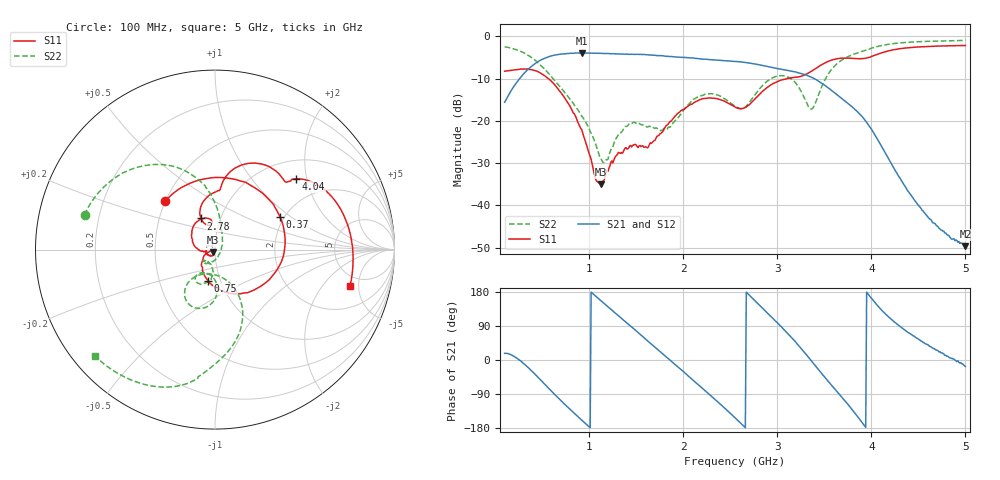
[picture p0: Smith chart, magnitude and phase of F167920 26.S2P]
!  2-Port S-parameters saved by WinCal
! VAR MeasName=S-Parameters (CALIBRATED_DATA) read from VNA (N5242A)
! VAR MeasDate=2016-11-22 9:56:27
! VAR NAME=F167920 26
! VAR FILENAME=F167920 26.S2P
! VAR DATE=2016-11-22 9:56:27
! VAR PHYS_PORTS=1,2
# Hz S DB R 50
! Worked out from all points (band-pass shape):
!   491 points, 100 MHz to 5 GHz, reference 50 ohm
!   highest |S21| = -3.91 dB at 920 MHz (marker M1); lowest = -49.7 dB at 5 GHz (marker M2)
!   |S21| within 3 dB of the highest: 396.6 MHz to 2.847 GHz (2.451 GHz wide, 151 % of centre)
!   lowest |S11| = -35.0 dB at 1.12 GHz (marker M3), VSWR 1.04, Z = 49 - j1.47 ohm
!   |S11| at or under -10 dB: 566.2 MHz to 3.101 GHz (2.535 GHz wide, 138 % of centre)
!   |S22| runs from -29.9 to -1.0 dB; largest |S21 - S12| = 0.0012
!   S11 on the Smith chart (normalised r, x): 100 MHz: 0.50, +0.32; 370 MHz: 1.90, +0.82; 750 MHz: 0.87, -0.31; 2.78 GHz: 0.81, +0.29; 4.04 GHz: 1.40, +1.73; 5 GHz: 3.86, -3.97
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1e8  -8.25 135.7  -15.60 17.5  -15.61 17.5  -2.47 165.1
2.3e8  -7.87 81.2  -10.85 4.7  -10.85 4.8  -3.20 145.9
3.7e8  -7.85 26.5  -7.40 -24.6  -7.40 -24.5  -4.76 124.9
5.6e8  -9.93 -42.3  -4.90 -72.4  -4.90 -72.4  -8.58 100.4
7.5e8  -14.99 -102.2  -4.10 -119.5  -4.09 -119.5  -13.55 85.1
9.2e8  -22.07 -146.0  -3.91 -158.6  -3.91 -158.6  -18.92 71.4
1.12e9  -35.02 -122.2  -4.02 157.3  -4.01 157.3  -28.75 10.7
1.18e9  -32.06 -102.9  -4.07 144.5  -4.07 144.5  -29.17 -42.0
1.43e9  -25.92 -144.0  -4.26 91.6  -4.26 91.6  -20.58 -122.8
1.74e9  -23.46 -172.4  -4.55 25.0  -4.55 25.0  -22.14 -126.9
1.94e9  -18.25 166.6  -4.92 -17.6  -4.92 -17.7  -19.43 -97.9
2.17e9  -15.05 133.1  -5.31 -67.7  -5.31 -67.8  -14.21 -106.4
2.36e9  -14.74 106.0  -5.64 -109.0  -5.65 -109.0  -13.87 -121.9
2.55e9  -16.75 96.7  -5.93 -152.2  -5.93 -152.2  -16.53 -120.0
2.78e9  -14.39 114.2  -6.61 152.1  -6.62 152.0  -13.30 -86.3
3.06e9  -10.24 94.8  -7.87 83.3  -7.89 83.4  -9.32 -111.9
3.37e9  -8.16 82.8  -9.74 -4.6  -9.75 -4.6  -17.12 -92.0
3.62e9  -5.37 62.7  -13.54 -79.2  -13.57 -79.0  -6.77 -71.7
4.04e9  -4.45 41.1  -23.39 151.2  -23.42 151.4  -2.54 -99.9
4.19e9  -3.39 32.2  -29.24 112.2  -29.30 112.5  -1.84 -108.7
4.6e9  -2.39 5.5  -42.71 40.3  -42.92 39.8  -1.18 -126.8
5e9  -2.16 -15.0  -49.66 -17.1  -49.64 -13.2  -0.97 -138.5
